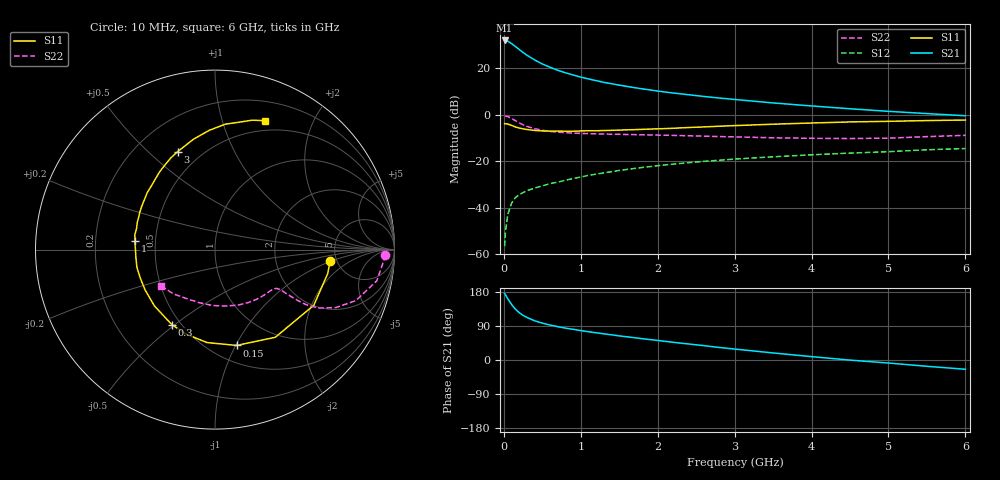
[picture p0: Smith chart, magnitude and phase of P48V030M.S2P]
! SIEMENS Small Signal Semiconductors
! BFP182
! Si NPN RF Bipolar Junction Transistor in SOT143
! VCE = 8 V  IC = 30 mA
! Common Emitter S-Parameters:  March  1996
# GHz  S  MA  R  50
!  f  S11  S21  S12  S22
! GHz  MAG  ANG  MAG  ANG  MAG  ANG  MAG  ANG
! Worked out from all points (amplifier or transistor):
!   36 points, 10 MHz to 6 GHz, reference 50 ohm
!   highest |S21| = 31.9 dB at 10 MHz (marker M1)
!   |S21| within 3 dB of that: start of sweep to 166.1 MHz
!   unconditionally stable (mu >= 1): 698.9 MHz to 5.677 GHz
!   at 250 MHz: K = 0.54, MSG = 30.1 dB, |S12| = -33.4 dB
!   at 1.4 GHz: K = 1.17, MAG = 16.4 dB, |S12| = -24.5 dB
!   at 6 GHz: K = 0.97, MSG = 7.0 dB, |S12| = -14.5 dB
!   S11 on the Smith chart (normalised r, x): 10 MHz: 4.42, -0.95; 150 MHz: 0.66, -1.01; 300 MHz: 0.45, -0.49; 1 GHz: 0.38, +0.04; 3 GHz: 0.37, +0.62; 6 GHz: 0.39, +1.39
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0.01  0.645 -5.6  39.53 175.5  0.0015 82.2  0.9476 -1.8
0.02  0.6421 -12.0  39.5 172.6  0.0029 79.9  0.9404 -4.2
0.05  0.6318 -29.4  38.2 161.9  0.0071 78.5  0.9182 -10.9
0.1  0.5928 -55.5  33.86 146.6  0.0125 64.6  0.8347 -19.9
0.15  0.5473 -77.3  29.35 134.2  0.0166 60.4  0.7469 -25.6
0.2  0.5198 -94.9  25.3 124.9  0.0191 55.3  0.67 -29.1
0.25  0.4977 -108.8  21.77 117.7  0.0213 53.2  0.6096 -30.9
0.3  0.4823 -119.9  19.08 112.3  0.0233 52.3  0.5626 -31.5
0.4  0.4608 -137.1  15.09 103.5  0.0266 52.4  0.501 -31.7
0.5  0.4497 -150.1  12.34 97.3  0.0296 52.4  0.4639 -31.7
0.6  0.4456 -159.4  10.52 92.2  0.0331 53.1  0.4398 -31.5
0.7  0.4462 -167.2  9.031 88.0  0.0357 54.0  0.4243 -31.6
0.8  0.4429 -174.0  8.004 84.1  0.039 54.5  0.4124 -31.9
1  0.4491 174.1  6.443 77.6  0.0459 55.1  0.3977 -33.2
1.1  0.454 169.4  5.894 74.6  0.0499 55.1  0.393 -34.2
1.5  0.4679 153.5  4.332 63.6  0.0636 54.0  0.38 -38.9
2.2  0.512 131.1  2.938 46.7  0.0869 49.4  0.3605 -50.5
3  0.5846 110.8  2.134 28.9  0.1116 42.2  0.335 -67.2
3.5  0.6267 101.0  1.795 18.6  0.125 37.5  0.32 -79.4
4.5  0.7013 85.3  1.346 -0.3  0.15 28.9  0.3082 -106.4
5.5  0.75 74.0  1.06 -16.6  0.1769 21.1  0.3389 -133.3
6  0.7711 68.7  0.952 -24.5  0.1881 16.2  0.3615 -146.1
